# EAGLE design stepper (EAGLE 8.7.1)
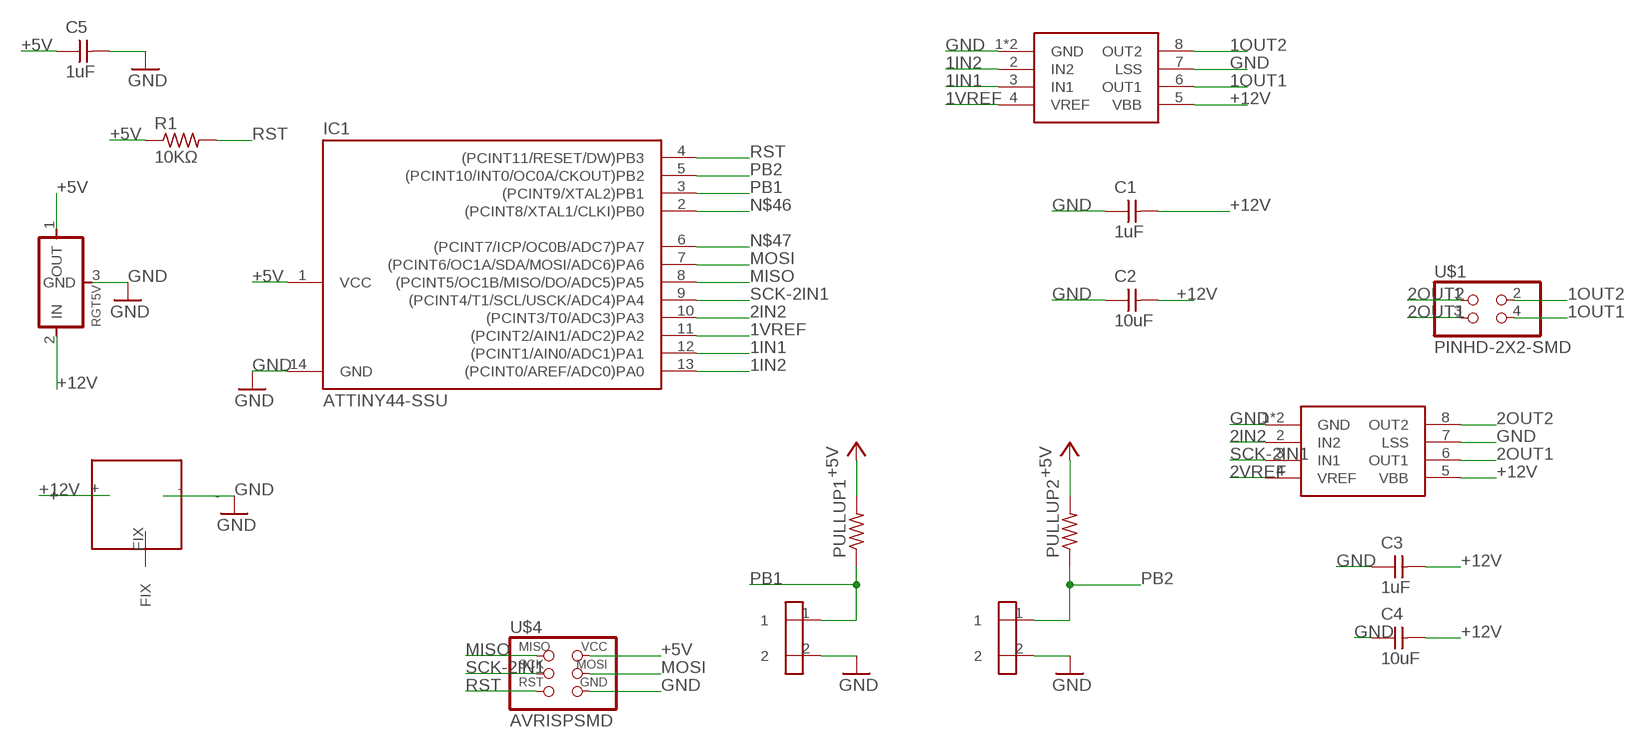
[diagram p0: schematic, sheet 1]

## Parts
C1  1uF  CAP-UNPOLARIZEDFAB  [C1206FAB]
C2  10uF  CAP-UNPOLARIZEDFAB  [C1206FAB]
C3  1uF  CAP-UNPOLARIZEDFAB  [C1206FAB]
C4  10uF  CAP-UNPOLARIZEDFAB  [C1206FAB]
C5  1uF  CAP-UNPOLARIZEDFAB  [C1206FAB]
DCJACK1  AKIZUKI_DCJACK  [AKIZUKI_DCJACK]
IC1  ATTINY44-SSU  [SOIC14]
PULLUP1  RES-US1206FAB  [R1206FAB]
PULLUP2  RES-US1206FAB  [R1206FAB]
R1  10KΩ  RES-US1206FAB  [R1206FAB]
RGT5V  REGULATORSOT23  [SOT23]
TML1  AKIZUKITNK_HOLE2PIN  [5.08PICH_HL]
TML2  AKIZUKITNK_HOLE2PIN  [5.08PICH_HL]
U$1  PINHD-2X2-SMD  [2X02SMD]
U$2  A4953-H-BRIDGE-MOTOR-DRIVER-PAD  [SOIC8_PAD]
U$3  A4953-H-BRIDGE-MOTOR-DRIVER-PAD  [SOIC8_PAD]
U$4  AVRISPSMD  [2X03SMD]

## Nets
1IN1: IC1.12((PCINT1/AIN0/ADC1)PA1) U$3.3(IN1)
1IN2: IC1.13((PCINT0/AREF/ADC0)PA0) U$3.2(IN2)
1OUT1: U$1.4 U$3.6(OUT1)
1OUT2: U$1.2 U$3.8(OUT2)
1VREF: IC1.11((PCINT2/AIN1/ADC2)PA2) U$3.4(VREF)
2IN2: IC1.10((PCINT3/T0/ADC3)PA3) U$2.2(IN2)
2OUT1: U$1.3 U$2.6(OUT1)
2OUT2: U$1.1 U$2.8(OUT2)
2VREF: U$2.4(VREF)
+5V: C5.1 IC1.1(VCC) PULLUP1.2 PULLUP2.2 R1.1 RGT5V.1(OUT) U$4.2(VCC)
+12V: C1.2 C2.2 C3.2 C4.2 DCJACK1.+ RGT5V.2(IN) U$2.5(VBB) U$3.5(VBB)
GND: C1.1 C2.1 C3.1 C4.1 C5.2 DCJACK1.- IC1.14(GND) RGT5V.3(GND) TML1.2 TML2.2 U$2.1(GND) U$2.7(LSS) U$2.GND U$3.1(GND) U$3.7(LSS) U$3.GND U$4.6(GND)
MISO: IC1.8((PCINT5/OC1B/MISO/DO/ADC5)PA5) U$4.1(MISO)
MOSI: IC1.7((PCINT6/OC1A/SDA/MOSI/ADC6)PA6) U$4.4(MOSI)
N$46: IC1.2((PCINT8/XTAL1/CLKI)PB0)
N$47: IC1.6((PCINT7/ICP/OC0B/ADC7)PA7)
PB1: IC1.3((PCINT9/XTAL2)PB1) PULLUP1.1 TML1.1
PB2: IC1.5((PCINT10/INT0/OC0A/CKOUT)PB2) PULLUP2.1 TML2.1
RST: IC1.4((PCINT11/RESET/DW)PB3) R1.2 U$4.5(RST)
SCK-2IN1: IC1.9((PCINT4/T1/SCL/USCK/ADC4)PA4) U$2.3(IN1) U$4.3(SCK)
Unconnected: DCJACK1.FIX

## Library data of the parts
C1-C5 = fab:CAP-UNPOLARIZED
DCJACK1 = doyo:AKIZUKI_DCJACK
IC1 = fab:ATTINY44
PULLUP1 PULLUP2 = fab:RES-US: Resistor (US Symbol)
R1 = HelloKamakura:RES-US: Resistor (US Symbol)
RGT5V = fab:REGULATOR
TML1 TML2 = doyo:AKIZUKI?TNK_HOLE2PIN
U$1 = fab:PINHD-2X2-SMD
U$2 U$3 = fab:A4953-H-BRIDGE-MOTOR-DRIVER-PAD
U$4 = HelloKamakura:AVRISP

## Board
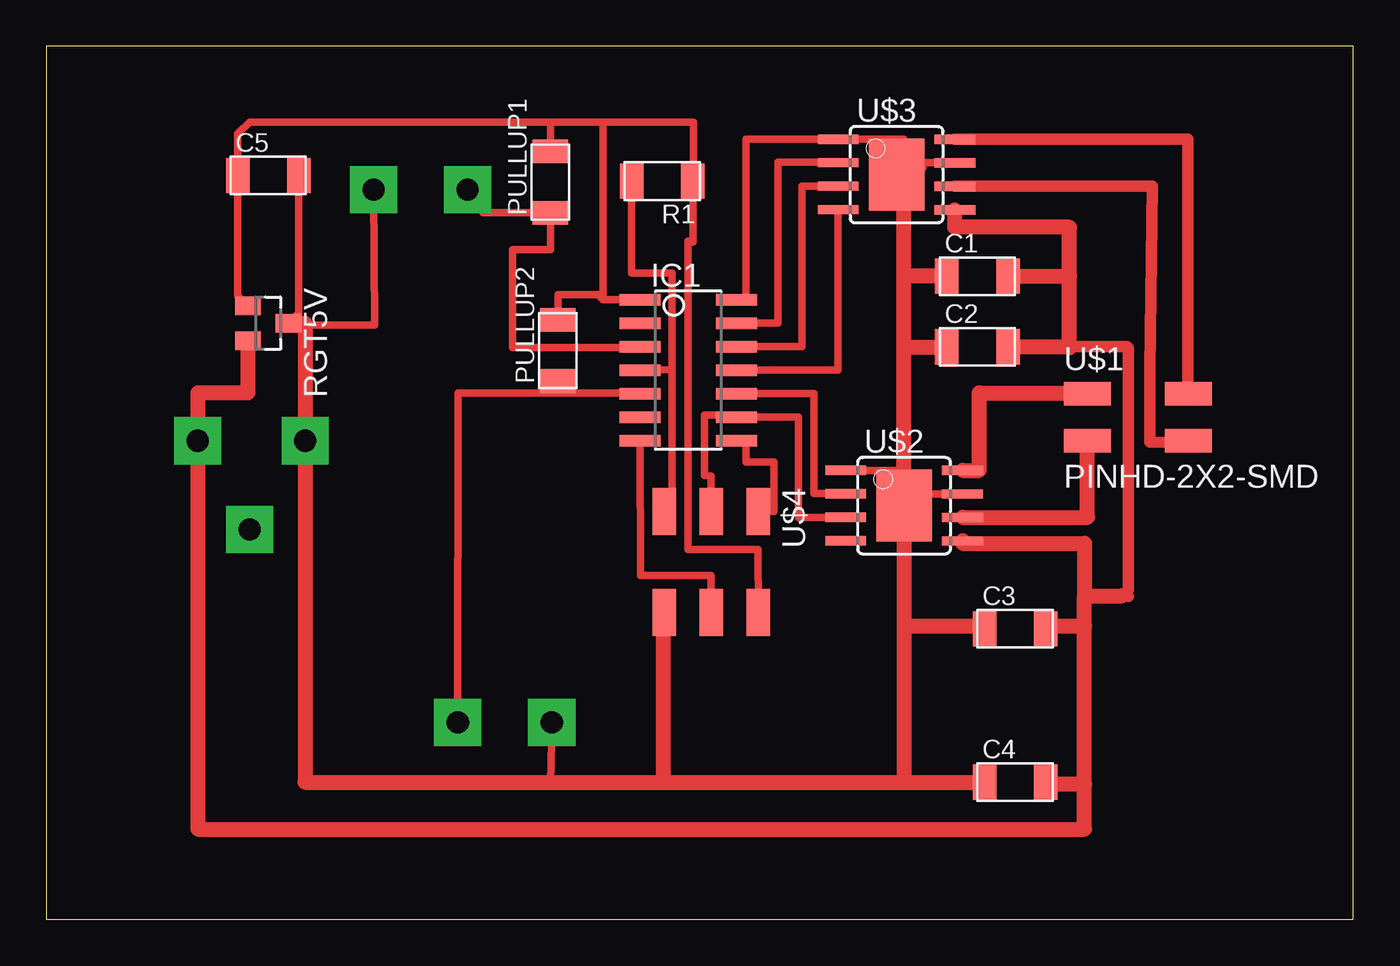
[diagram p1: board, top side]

Size 70.59 x 47.17 mm. Coordinates in mm from the lower left corner, seen from the top.
Outline: 0,0 70.59,0 70.59,47.17 0,47.17 0,0
Copper layers (1*16): Top 0.035mm / dielectric 1.5mm / Bottom 0.035mm
Design rules "default *": minimum track width 6mil, minimum drill 0.35mm, track to track 0.4mm, track to pad 0.4mm, pad to pad 0.4mm, via to via 0.4mm, smd to smd 0.4mm, copper to edge 40mil, drill to drill 6mil, minimum pad ring 10mil, minimum via ring 8mil, stop-mask expansion 4mil, vias tented up to drill 0mil, thermal gap 10mil

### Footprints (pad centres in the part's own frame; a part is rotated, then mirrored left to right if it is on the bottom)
C1206FAB = smd 1.27 x 1.905: 1 -1.651,0; 2 1.651,0
AKIZUKI_DCJACK = drill 1.2 pad 2.54 square: + 0,0; - 0,5.8; FIX 4.8,2.8
SOIC14 = smd 0.61 x 2.21: 1 -3.81,-2.603; 2 -2.54,-2.603; 3 -1.27,-2.603; 4 0,-2.603; 5 1.27,-2.603; 6 2.54,-2.603; 7 3.81,-2.603; 8 3.81,2.603; 9 2.54,2.603; 10 1.27,2.603; 11 0,2.603; 12 -1.27,2.603; 13 -2.54,2.603; 14 -3.81,2.603
R1206FAB = smd 1.27 x 1.905: 1 -1.651,0; 2 1.651,0
SOT23 = smd 1 x 1.4: 1 -0.95,-1.1; 2 0.95,-1.1; 3 0,1.1
5.08PICH_HL = drill 1.2 pad 2.54 square: 1 0,0; 2 -5.08,0
2X02SMD = smd 2.54 x 1.27: 1 -2.54,1.27; 2 2.92,1.27; 3 -2.54,-1.27; 4 2.92,-1.27
SOIC8_PAD = smd 0.5 x 2.2: 1 -1.905,-3.154; 2 -0.645,-3.154; 3 0.625,-3.154; 4 1.895,-3.154; 5 1.905,3.154; 6 0.635,3.154; 7 -0.635,3.154; 8 -1.905,3.154 | smd 3.886 x 2.997: GND 0,0
2X03SMD = smd 2.54 x 1.27: 1 -2.54,2.54; 2 2.92,2.54; 3 -2.54,0; 4 2.92,0; 5 -2.54,-2.54; 6 2.92,-2.54

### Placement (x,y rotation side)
C1  50.29,34.75 0 top
C2  50.29,30.94 0 top
C3  52.32,15.7 0 top
C4  52.32,7.42 0 top
C5  11.99,40.18 0 top
DCJACK1  8.18,25.86 270 top
IC1  34.67,29.67 270 top
PULLUP1  27.23,39.83 90 top
PULLUP2  27.64,30.73 90 top
R1  33.27,39.88 180 top
RGT5V  11.99,32.21 270 top
TML1  22.76,39.42 0 top
TML2  22.23,10.64 180 top
U$1  58.78,27.13 0 top
U$2  46.33,22.35 270 top
U$3  45.92,40.23 270 top
U$4  35.92,19.51 270 top

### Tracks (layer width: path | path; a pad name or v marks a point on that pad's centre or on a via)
1IN1
  Top 0.406: IC1.12 40.82,30.94 40.82,39.6 42.77,39.6 U$3.3
1IN2
  Top 0.406: IC1.13 39.52,32.21 39.52,40.92 42.77,40.92 U$3.2
1OUT1
  Top 0.61: U$3.6 59.74,39.6 59.61,29.74 59.59,29.76 59.59,25.78 62.2,25.76 62.2,25.73 61.7,25.73 U$1.4
1OUT2
  Top 0.61: U$3.8 61.67,42.14 61.67,28.4 61.77,28.4
  Top 0.813: 61.77,28.4 U$1.2
1VREF
  Top 0.406: U$3.4 42.77,29.67 IC1.11
2IN2
  Top 0.406: IC1.10 41.45,28.4 41.45,23 U$2.2
2OUT1
  Top 0.813: U$2.6 56.24,21.72 U$1.3
2OUT2
  Top 0.813: U$2.8 50.39,24.26 50.39,28.45 56.24,28.45 U$1.1
+5V
  Top 0.406: 27.23,43.08 10.97,43.08 10.34,42.44 C5.1 10.34,33.71 RGT5V.1 | 27.23,43.08 30.07,43.08 | 30.07,43.08 34.95,43.08 34.95,39.9 R1.1 34.92,36.58 34.67,36.65 34.67,19.99 38.43,19.99 | 38.43,19.99 38.43,19.94 | 38.43,19.99 U$4.2 | IC1.1 30.07,33.48 | 30.07,33.48 30.07,43.08 | PULLUP1.2 27.23,43.08 | 30.07,33.48 29.79,33.76 27.64,33.76 PULLUP2.2
+12V
  Top 0.61: 58.45,17.45 58.12,17.48 58.45,17.8 58.45,30.86 58.37,30.94 54.86,30.94
  Top 0.813: RGT5V.2 10.89,28.45 8.18,28.45 DCJACK1.+ 8.18,4.88 56.08,4.88 56.08,7.32 | 55.27,30.94 55.27,34.75 | 55.27,34.75 55.27,37.39 49.08,37.39 U$3.5 | C2.2 54.86,30.94 55.27,30.94 | 55.27,30.94 55.27,30.89 | C1.2 55.27,34.75 | 56.08,7.32 56.08,15.85 | 56.08,15.85 56.08,17.48 | 56.08,17.48 58.12,17.48 | C3.2 53.98,15.85 56.08,15.85 | C4.2 53.98,7.32 56.08,7.32 | U$2.5 49.48,20.32 56.08,20.32 56.08,17.48
GND
  Top 0.406: C5.2 13.64,32.76 RGT5V.3 | U$2.7 47.14,22.99 47.14,22.76 46.33,22.76 46.33,23.16 | U$2.1 46.33,24.26 46.33,23.57 | U$3.7 46.33,40.87 | 46.33,40.87 46.33,40.64 | 46.33,40.87 46.33,42.14 U$3.1 37.8,42.14 37.8,33.48 IC1.14 | 13.98,32.21 14.08,32.11 17.73,32.11 TML1.2 | TML2.2 27.23,7.42
  Top 0.813: RGT5V.3 13.98,32.21 DCJACK1.- 13.98,7.42 27.23,7.42 33.33,7.42 | 33.33,7.42 46.33,7.42 | 46.33,7.42 C4.1 | U$4.6 33.33,16.59 33.33,7.42 | C2.1 48.64,30.89 46.33,30.89 | 46.33,15.85 U$2.GND 46.33,23.16 46.33,23.57 46.33,30.89 | 46.33,15.85 46.33,7.42 | 46.33,30.89 46.33,34.75 | 46.33,34.75 46.33,40.64 47.14,40.64 U$3.GND | C1.1 46.33,34.75 | 46.33,15.85 50.67,15.85 C3.1
MISO
  Top 0.406: IC1.8 37.8,25.86 37.8,24.71 39.29,24.71 39.29,22.05 U$4.1
MOSI
  Top 0.406: IC1.7 32.09,18.57 35.92,18.57 U$4.4
PB1
  Top 0.406: TML1.1 23.6,38.18 PULLUP1.1 27.23,36.17 25.2,36.17 25.2,30.89 32.07,30.89 IC1.3
PB2
  Top 0.406: IC1.5 32.07,28.45 27.64,28.45 | 27.64,28.45 PULLUP2.1 | 27.64,28.45 22.25,28.45 TML2.1
RST
  Top 0.406: R1.2 31.62,34.92 33.8,34.92 33.8,29.69 | 33.8,29.69 33.8,22.07 U$4.5 | IC1.4 33.8,29.69
SCK-2IN1
  Top 0.406: U$2.3 43.18,21.72 40.64,21.72 40.64,27.13 IC1.9 37.16,27.24 36.58,27.24 | 37.3,27.23 36.58,27.24 | 36.58,27.24 35.54,27.25 35.54,23.98 35.92,23.95 U$4.3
